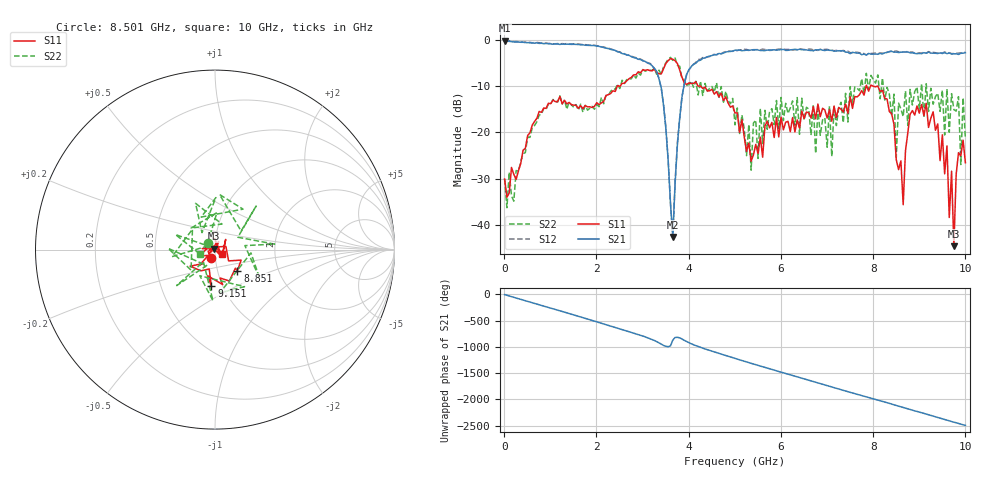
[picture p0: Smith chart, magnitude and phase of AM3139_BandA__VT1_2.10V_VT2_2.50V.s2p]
! Date/Time: Tue, Nov 13, 2018 4:57 PM
! Network Analyzer: Agilent Technologies E8364B Rev: A.07.50.67
! Sweep from 0.010 to 10.000 GHz, 201 Points, Sweep Type: LIN
! Power Supply: 2.101 V, 0.000 A
# Hz S DB R 50
!freq MagS11 AngS11 MagS21 AngS21 MagS12 AngS12 MagS22 AngS22
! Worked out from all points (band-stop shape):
!   201 points, 10 MHz to 10 GHz, reference 50 ohm
!   highest |S21| = -0.26 dB at 10 MHz (marker M1); lowest = -42.6 dB at 3.656 GHz (marker M2)
!   |S21| within 3 dB of the highest: start of sweep to 2.65 GHz; 4.589 GHz to 7.752 GHz (3.163 GHz wide, 51.3 % of centre)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
!   lowest |S11| = -44.6 dB at 9.75 GHz (marker M3), VSWR 1.01, Z = 49.6 + j0.443 ohm
!   |S11| at or under -10 dB: start of sweep to 2.453 GHz; 4.256 GHz to 7.849 GHz (3.593 GHz wide, 59.4 % of centre); 7.991 GHz to end of sweep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
!   |S22| runs from -36.3 to -3.8 dB; largest |S21 - S12| = 0.03
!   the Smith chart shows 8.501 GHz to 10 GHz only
!   S11 on the Smith chart (normalised r, x): 8.501 GHz: 0.95, -0.08; 8.851 GHz: 1.25, -0.30; 9.151 GHz: 0.89, -0.38; 10 GHz: 1.08, -0.05
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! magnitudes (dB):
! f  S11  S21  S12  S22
! 10 MHz  -30.1  -0.3  -0.2  -30.1
! 1.708 GHz  -14.9  -1.1  -1.0  -15.7
! 3.357 GHz  -7.4  -8.5  -8.4  -6.6
! 3.656 GHz  -4.2  -42.6  -42.7  -4.5
! 3.956 GHz  -9.7  -7.5  -7.6  -9.8
! 5.005 GHz  -15.8  -2.3  -2.4  -18.4
! 5.355 GHz  -26.2  -2.2  -2.2  -28.2
! 5.554 GHz  -21.1  -2.4  -2.2  -14.9
! 6.703 GHz  -14.5  -2.4  -2.2  -14.0
! 7.103 GHz  -17.6  -2.3  -2.3  -25.2
! 7.502 GHz  -12.3  -3.0  -2.8  -10.1
! 8.352 GHz  -15.5  -2.6  -2.6  -11.8
! 8.501 GHz  -25.9  -2.7  -2.4  -25.4
! 8.651 GHz  -35.6  -2.7  -2.7  -16.6
! 8.851 GHz  -15.3  -2.8  -2.7  -14.1
! 9.151 GHz  -13.7  -2.9  -2.9  -9.5
! 9.6 GHz  -22.9  -3.0  -2.9  -10.7
! 9.75 GHz  -44.6  -3.1  -3.0  -15.1
! 9.85 GHz  -24.4  -3.2  -2.9  -12.3
! 9.9 GHz  -25.1  -3.0  -2.9  -26.9
! 9.95 GHz  -21.7  -2.9  -2.8  -12.5
! 10 GHz  -26.6  -2.8  -2.7  -21.4
